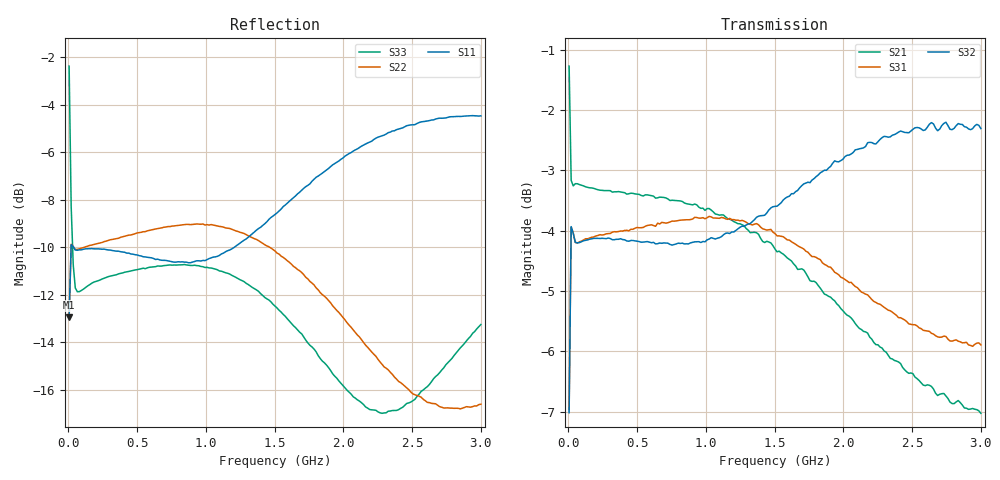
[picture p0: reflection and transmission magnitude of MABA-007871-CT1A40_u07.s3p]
#	MHz	S	RI	R	50
!FREQ	R1	I1	R2	I2	R3	I3
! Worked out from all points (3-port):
!   201 points, 5 MHz to 3 GHz, reference 50 ohm
!   strongest paths, dB at 5 MHz, 753.8 MHz, 1.502 GHz, 2.251 GHz, 3 GHz:
!     S32: -7.0, -4.2, -3.6, -2.5, -2.3
!     S31: -7.0, -3.8, -4.0, -5.2, -5.9
!     S21: -1.3, -3.5, -4.3, -5.9, -7.0
!   lowest |S11| = -12.9 dB at 5 MHz (marker M1), VSWR 1.58, Z = 64.3 + j22 ohm
!   |S11| at or under -10 dB: start of sweep to 19.44 MHz; 37.45 MHz to 1.207 GHz (1.169 GHz wide, 188 % of centre)
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5  0.156 0.1624  0.8452 -0.1688  -0.3101 -0.3242
   0.8468 -0.1688  0.153 0.1637  0.3077 0.3253
   -0.3101 -0.3242  0.3044 0.3257  -0.3854 0.6548
19.975  0.3138 0.0636  0.6885 -0.0898  -0.621 -0.1338
        0.6884 -0.0905  0.3119 0.0748  0.6191 0.1449
        -0.621 -0.1338  0.619 0.1447  0.2443 0.2978
34.95  0.3168 0.0135  0.6845 -0.0601  -0.6267 -0.0399
       0.6845 -0.0603  0.3156 0.0328  0.6252 0.0589
       -0.6267 -0.0399  0.625 0.059  0.2583 0.1326
439.275  0.212 -0.2226  0.5976 -0.3217  -0.5622 0.2858
         0.5972 -0.3187  0.3345 -0.0232  0.6174 -0.0495
         -0.5622 0.2858  0.6164 -0.0483  0.2809 0.0141
798.675  -0.0104 -0.2946  0.4123 -0.5282  -0.4084 0.4969
         0.4153 -0.523  0.3421 -0.0808  0.6106 -0.0857
         -0.4084 0.4969  0.6099 -0.0866  0.2894 -0.0219
1143.1  -0.241 -0.1941  0.1509 -0.6292  -0.1801 0.6196
        0.162 -0.627  0.3133 -0.1496  0.6171 -0.1136
        -0.1801 0.6196  0.617 -0.1152  0.2722 -0.0632
1502.5  -0.3644 0.0668  -0.1336 -0.5869  0.082 0.6221
        -0.1205 -0.5971  0.2407 -0.1962  0.6458 -0.1592
        0.082 0.6221  0.6409 -0.1609  0.2213 -0.0874
1816.975  -0.3068 0.3241  -0.3202 -0.4492  0.2671 0.535
          -0.3194 -0.4699  0.1696 -0.1933  0.6715 -0.2285
          0.2671 0.535  0.6648 -0.224  0.1724 -0.0726
2251.25  -0.0272 0.538  -0.4405 -0.2013  0.4179 0.3558
         -0.4603 -0.2135  0.1115 -0.1462  0.6655 -0.3606
         0.4179 0.3558  0.6589 -0.3529  0.1415 -0.0169
3000  0.4682 0.371  -0.3967 0.1712  0.5034 0.063
      -0.4016 0.1922  0.118 -0.0891  0.5161 -0.5857
      0.5034 0.063  0.5127 -0.5699  0.2101 0.0565
